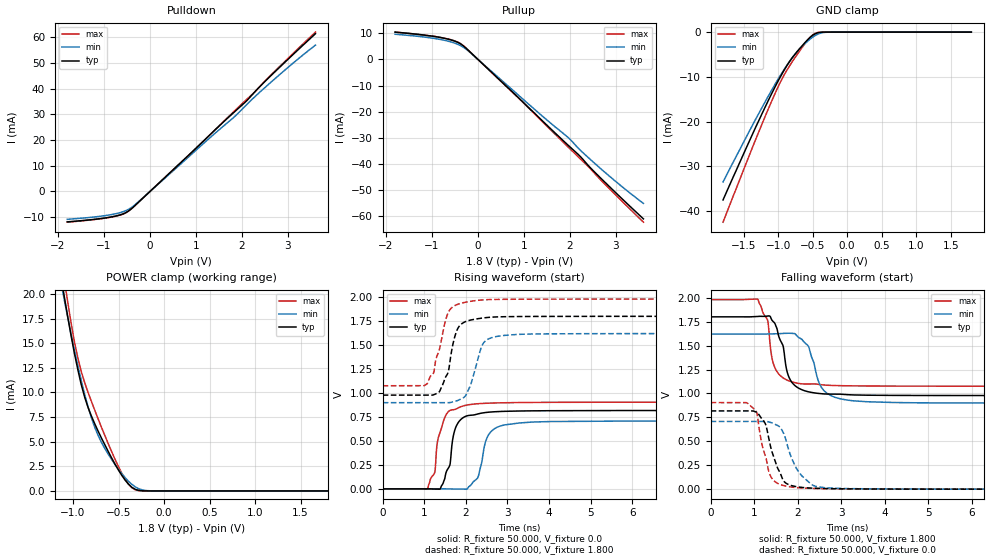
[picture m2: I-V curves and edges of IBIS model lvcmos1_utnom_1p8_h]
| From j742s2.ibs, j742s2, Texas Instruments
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|   utnom_1p8_h
[Model]   lvcmos1_utnom_1p8_h
Model_type I/O
Polarity   Non-Inverting
Enable   Active-High
Vinl = 0
Vinh = 0.8
Vmeas = 0.9
Vref = 1.8
Cref = 2pF
Rref = 100000
|   typ   min   max
C_comp   2.521pF   2.296pF   2.733pF
[Voltage Range]   1.8   1.62   1.98
[Temperature Range]   27   150   -40
[Pullup Reference]   1.8   1.62   1.98
[Pulldown Reference]   0   0   0
[Power Clamp Reference]   1.8   1.62   1.98
[GND Clamp Reference]   0   0   0
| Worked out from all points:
|   slope of the pulldown table from 0 to 0.27 V, typ, clamps not added: 59.6 ohm
|   slope of the pullup table from 0 to 0.27 V, typ, clamps not added: 60.3 ohm
|   GND clamp passes 1 mA (typ) near -0.52 V on its own axis
|   POWER clamp passes 1 mA (typ) near -0.42 V on its own axis
|   rising waveform, R_fixture 50.000, V_fixture 0.0: 20-80 % time 250ps typ, 243ps min, 219ps max; typ from 0 V to 0.817 V
|   rising waveform, R_fixture 50.000, V_fixture 1.800: 20-80 % time 280ps typ, 299ps min, 295ps max; typ from 0.978 V to 1.8 V
|   falling waveform, R_fixture 50.000, V_fixture 1.800: 20-80 % time 285ps typ, 318ps min, 223ps max; typ from 1.8 V to 0.978 V
|   falling waveform, R_fixture 50.000, V_fixture 0.0: 20-80 % time 324ps typ, 399ps min, 252ps max; typ from 0.817 V to 0 V
[Pulldown]
|Voltage   I(typ)   I(min)   I(max)
-1.8V     -11.83mA   -10.84mA   -11.95mA
-1.194V   -10.81mA   -9.89mA    -10.89mA
-808mV    -9.786mA   -8.891mA   -9.883mA
-588mV    -8.73mA    -7.88mA    -8.834mA
-422mV    -7.005mA   -6.479mA   -7.05mA
-257mV    -4.32mA    -4.115mA   -4.313mA
955mV     16.06mA    15.31mA    16.02mA
1.837V    30.98mA    29.08mA    31.32mA
2.057V    34.53mA    32.96mA    35.07mA
2.278V    38.73mA    36.83mA    38.74mA
2.718V    46.59mA    43.91mA    46.88mA
3.6V      61.43mA    56.98mA    62.05mA
[Pullup]
|Voltage   I(typ)   I(min)   I(max)
-1.8V     10.4mA     9.589mA    10.42mA
-808mV    8.34mA     7.569mA    8.342mA
-533mV    7.149mA    6.374mA    7.216mA
-367mV    5.814mA    5.164mA    5.926mA
-202mV    3.357mA    3.122mA    3.385mA
900mV     -14.95mA   -13.95mA   -15.06mA
1.947V    -32.54mA   -29.6mA    -33.21mA
2.222V    -37mA      -34.61mA   -37.92mA
2.443V    -41.33mA   -38.19mA   -41.71mA
2.718V    -46.16mA   -42.47mA   -46.9mA
3.214V    -54.57mA   -49.76mA   -55.58mA
3.6V      -60.94mA   -55.01mA   -62.2mA
[GND_clamp]
|Voltage   I(typ)   I(min)   I(max)
-1.8V     -37.5mA    -33.49mA   -42.48mA
-1.318V   -20.97mA   -19.21mA   -23.65mA
-1.132V   -14.92mA   -13.99mA   -16.76mA
-984mV    -10.42mA   -10.06mA   -11.66mA
-872mV    -7.442mA   -7.36mA    -8.464mA
-761mV    -5.052mA   -4.998mA   -5.817mA
-687mV    -3.663mA   -3.691mA   -4.162mA
-575mV    -1.728mA   -2.058mA   -1.807mA
-501mV    -716.8uA   -1.141mA   -632.9uA
-427mV    -157.5uA   -468.3uA   -83.58uA
-278mV    -1.328uA   -23.76uA   -249.6nA
1.8V      0A         0A         0A
[POWER_clamp]
|Voltage   I(typ)   I(min)   I(max)
-1.8V     63.27mA    56.65mA    71.18mA
-1.095V   19.71mA    19.39mA    21.45mA
-1.058V   17.7mA     17.64mA    19.19mA
-984mV    13.96mA    14.29mA    15.13mA
-946mV    12.28mA    12.71mA    13.48mA
-872mV    9.531mA    9.825mA    11mA
-761mV    6.815mA    6.464mA    8.201mA
-649mV    4.665mA    4.293mA    5.607mA
-464mV    1.58mA     1.753mA    1.804mA
-315mV    158.8uA    405.7uA    108.9uA
-130mV    309.5nA    7.673uA    148.4nA
1.8V      0A         0A         0A
[Ramp]
| variable   typ   min   max
dV/dt_r   0.490/0.250n   0.424/0.242n   0.543/0.219n
dV/dt_f   0.493/0.285n   0.432/0.315n   0.543/0.223n
R_load = 50.000
[Rising Waveform]
R_fixture= 50.000
V_fixture= 0.0
V_fixture_min= 0.0
V_fixture_max= 0.0
|time   V(typ)   V(min)   V(max)
0s        823.8nV    18.05uV    1.398uV
1.077ns   136.7uV    18.69uV    -890.4uV
1.255ns   -2.306mV   28.56uV    178.4mV
1.387ns   1.537mV    56.89uV    598.6mV
1.752ns   636.5mV    -1.598mV   830.2mV
2.013ns   759.8mV    -3.259mV   873.2mV
2.29ns    781.6mV    119.9mV    888.1mV
2.544ns   799.5mV    562.8mV    893.9mV
2.934ns   808.7mV    667.3mV    898.2mV
10ns      817.3mV    707.4mV    904.2mV
[Rising Waveform]
R_fixture= 50.000
V_fixture= 1.800
V_fixture_min= 1.620
V_fixture_max= 1.980
|time   V(typ)   V(min)   V(max)
0s        977.8mV    899.3mV    1.076V
1.069ns   977.9mV    899.3mV    1.096V
1.221ns   980.6mV    899.3mV    1.208V
1.363ns   1.014V     899.3mV    1.454V
1.584ns   1.235V     899.4mV    1.847V
1.757ns   1.62V      915.7mV    1.917V
1.992ns   1.745V     971.5mV    1.947V
2.403ns   1.782V     1.507V     1.971V
2.706ns   1.793V     1.587V     1.976V
10ns      1.8V       1.62V      1.98V
[Falling Waveform]
R_fixture= 50.000
V_fixture= 1.800
V_fixture_min= 1.620
V_fixture_max= 1.980
|time   V(typ)   V(min)   V(max)
0s        1.8V       1.62V      1.98V
1.086ns   1.804V     1.62V      1.983V
1.314ns   1.809V     1.621V     1.755V
1.362ns   1.807V     1.622V     1.53V
1.528ns   1.67V      1.623V     1.225V
1.781ns   1.191V     1.629V     1.134V
2.003ns   1.06V      1.591V     1.106V
2.544ns   997.1mV    1.064V     1.091V
2.977ns   992.4mV    943.8mV    1.081V
10ns      977.8mV    899.4mV    1.076V
[Falling Waveform]
R_fixture= 50.000
V_fixture= 0.0
V_fixture_min= 0.0
V_fixture_max= 0.0
|time   V(typ)   V(min)   V(max)
0s        817.3mV    707.5mV    904.3mV
825ps     817.3mV    707.5mV    903.8mV
1.084ns   792.1mV    707.5mV    739mV
1.266ns   672.8mV    707.5mV    334.4mV
1.359ns   481.5mV    699.2mV    155.1mV
1.591ns   174.7mV    648.4mV    49.83mV
1.738ns   60.24mV    499.7mV    31.52mV
2.052ns   20.85mV    163.2mV    13.31mV
2.497ns   7.87mV     22.14mV    6.191mV
10ns      33.03uV    87.62uV    16.22uV
